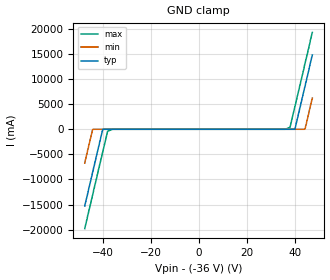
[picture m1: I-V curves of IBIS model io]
| TEXAS INSTRUMENTS INCORPORATED
| 2 Channel-Bi-directional ESD Protection Device
| Marketing Part #   Voltage Range   Package-type   #pins/pkg drawing
| ESD2CAN36-Q1   -36V-36V   SOT   3/DBZ
[IBIS Ver]   4.1
[Comment char]  |_char
[File Name]   esd2can36-q1.ibs
[File Rev]   1.0
"[Date]   Dec 20, 2023 "
[Source]   Data created from TI-SPICE simulations at TI-SLL/HVL.
   The following is an IBIS list for the TPD2E2U06.
   Please contact sllibis@ti.com with questions and
   comments concerning SLL IBIS models.
[Notes]   Revision_History:
   Rev 1.0: 6/12/2013
   - Initial release based on similar device
   Rev 2.0: 7/25/2013
   - New measurements under nominal conditions only.
[Disclaimer]
"| TI and its licensors and suppliers make no warranties, either expressed"
"| or implied, with respect to this  model, including the warranties of "
"| provided solely on an ""as is"" basis. The entire risk as to its quality "
| and performance is with the customer.
[Copyright]
| (C) Copyright 2023 Texas Instruments Incorporated. All rights reserved.
| Component ESD2CAN36-Q1_DBZ 3-PIN SOT
[Component]   ESD2CAN36-Q1_DBZ
"[Manufacturer]   Texas Instruments, Inc."
[Package]   |3 SOT - DBZ package
   typ   min   max
R_pkg   70.0E-03   60.0E-03   80.0E-03
L_pkg   5.0E-10   2.50E-10   10.0E-10
C_pkg   4.5E-13   2.50E-13   6.50E-13
[Pin]   signal_name   model_name   R_pin   L_pin   C_pin
1   IO   io   2.07E-03   2.09E-10   6.95E-14
2   IO   io   2.07E-03   2.09E-10   6.95E-14
3   GND   gnd   2.07E-03   2.09E-10   6.95E-14
| Models and submodels in the file (1): io (Input)
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|   io Model
[Model]   io
Model_type  Input
| variable   typ   min   max
C_comp   2.8pF   2.1pF   3.5pF
[Voltage Range]   72   68   76
[Temperature Range]   27   -55   150
[Power Clamp Reference]   0   0   0
[GND Clamp Reference]   -36   -34   -38
[GND Clamp]
|	Voltage  I(typ)   I(min)   I(max)
-47.5V    -15.3A     -6.73A     -19.8A
-44.3V    -8.67A     -102mA     -13.2A
-40V      -10nA      -10nA      -4.49A
-38V      -9.5nA     -9.5nA     -408mA
-36V      -9nA       -9nA       -9nA
36V       9nA        9nA        9nA
38V       9.5nA      9.5nA      408mA
40V       10nA       10nA       4.49A
44.3V     8.67A      102mA      13.2A
46.3V     12.8A      4.18A      17.2A
46.5V     13.3A      4.69A      17.8A
47.3V     14.8A      6.22A      19.3A
[Power Clamp]
|   Voltage   I(typ)   I(min)   I(max)
-36V      0A         0A         0A
0V        0A         0A         0A
36V       0A         0A         0A
